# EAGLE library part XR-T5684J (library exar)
T1 LINE INTERFACE
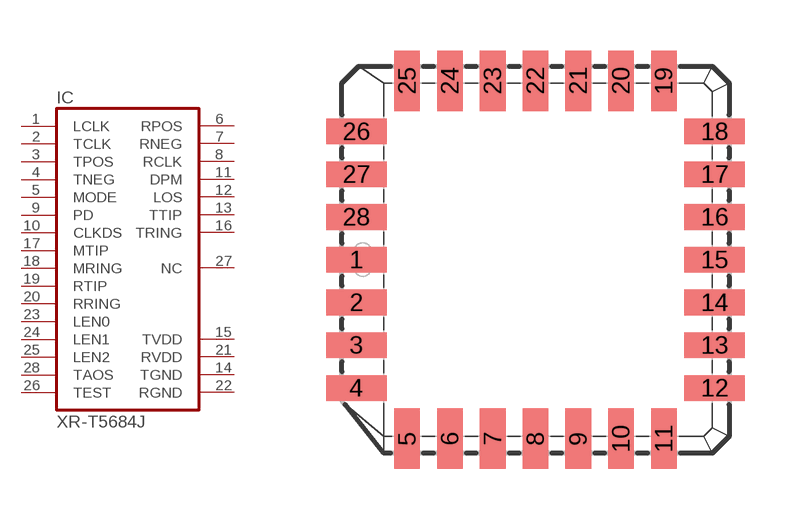
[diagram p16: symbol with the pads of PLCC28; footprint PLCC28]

Designator prefix IC

## XR-T5684J (OC_FARNELL: unknown; OC_NEWARK: unknown)  [PLCC28]
1  LCLK  in
2  TCLK  in
3  TPOS  in
4  TNEG  in
5  MODE  in
6  RPOS  out
7  RNEG  out
8  RCLK  out
9  PD  in
10  CLKDS  in
11  DPM  out
12  LOS  out
13  TTIP  out
14  TGND  pwr
15  TVDD  pwr
16  TRING  out
17  MTIP  in
18  MRING  in
19  RTIP  in
20  RRING  in
21  RVDD  pwr
22  RGND  pwr
23  LEN0  in
24  LEN1  in
25  LEN2  in
26  TEST  in
27  NC  nc
28  TAOS  in

## Footprint PLCC28 (pad centres in mm)
Plastic Leaded Chip Carrier
smd 1.8 x 0.76: 1 -5.32,0; 2 -5.32,-1.27; 3 -5.32,-2.54; 4 -5.32,-3.81; 12 5.32,-3.81; 13 5.32,-2.54; 14 5.32,-1.27; 15 5.32,0; 16 5.32,1.27; 17 5.32,2.54; 18 5.32,3.81; 26 -5.32,3.81; 27 -5.32,2.54; 28 -5.32,1.27
smd 0.76 x 1.8: 5 -3.81,-5.32; 6 -2.54,-5.32; 7 -1.27,-5.32; 8 0,-5.32; 9 1.27,-5.32; 10 2.54,-5.32; 11 3.81,-5.32; 19 3.81,5.32; 20 2.54,5.32; 21 1.27,5.32; 22 0,5.32; 23 -1.27,5.32; 24 -2.54,5.32; 25 -3.81,5.32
